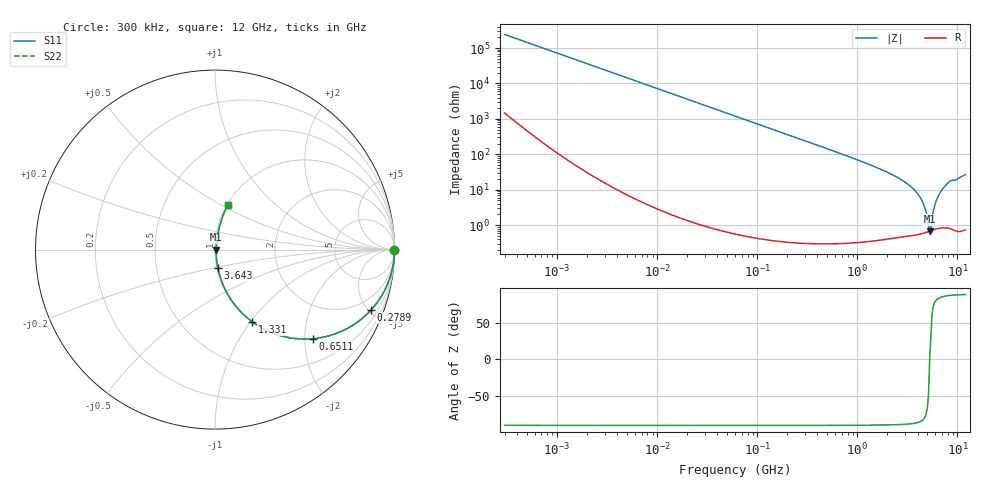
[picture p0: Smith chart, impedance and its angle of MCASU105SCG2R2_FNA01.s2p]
! MCASU105SCG2R2_FNA01  S-PARAMETER MODEL  ( Standard Model )
! Model Generated by TAIYO YUDEN Corporation (http://www.ty-top.com)
! Version 1.0
! TAIYO YUDEN Control No. 230609
! Copyright(c) 2023 TAIYO YUDEN CO.,LTD. All Rights Reserved.
! Product Description (link to TY-COMPAS)
! https://ds.yuden.co.jp/TYCOMPAS/or/detail?pn=MCASU105SCG2R2CFNA01&u=M
! Products Name : Multilayer Ceramic Capacitors
! Characteristics :
!  Capacitance : 2.2 [pF] , Rated Voltage : 50 [V] , TCC : CG / C0G
!  Case Size : 1.0 x 0.5 / 0.039 x 0.02 [mm/inch] , Thickness : 0.5 / 0.02 [mm/inch]
!  (Conditions: Temperature = 25 [degC] , DC Bias Voltage = 0 [V])
! External Node Assignments :
!  1  o---| |---o  2
! GND o---------o GND
! Frequency Range : 0.3MHz  -  12000MHz  [ 401 STEP ]
# MHZ S RI R 50
! Freq[MHz].  S11 Real  S11 Imag  S21 Real  S21 Imag  S12 Real  S12 Imag  S22 Real  S22 Imag
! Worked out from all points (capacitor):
!   401 points, 300 kHz to 12 GHz, reference 50 ohm
!   read as one part in series: C = 2.2 pF near 316.3 kHz
!   lowest |Z| = 674 mohm at 5.279 GHz (marker M1)
!   series resonance near 5.278 GHz, so ESL is about 410 pH
!   S11 on the Smith chart (normalised r, x): 300 kHz: open; 278.9 MHz: 1.01, -5.17; 651.1 MHz: 1.01, -2.19; 1.331 GHz: 1.01, -1.02; 3.643 GHz: 1.01, -0.21; 12 GHz: 1.01, +0.53
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0.3  1 -0.000415  2.68e-06 0.000415  2.68e-06 0.000415  1 -0.000415
1.769972  1 -0.00245  8.24e-06 0.00245  8.24e-06 0.00245  1 -0.00245
10.44266  0.9998 -0.0144  0.000214 0.0144  0.000214 0.0144  0.9998 -0.0144
60  0.9931 -0.0824  0.00687 0.0824  0.00687 0.0824  0.9931 -0.0824
278.9009  0.8697 -0.3361  0.1303 0.3361  0.1303 0.3361  0.8697 -0.3361
353.9943  0.8051 -0.3954  0.1949 0.3954  0.1949 0.3954  0.8051 -0.3954
651.0506  0.5448 -0.4966  0.4552 0.4966  0.4552 0.4966  0.5448 -0.4966
1331.232  0.2073 -0.402  0.7927 0.402  0.7927 0.402  0.2073 -0.402
2088.533  0.0818 -0.2671  0.9182 0.2671  0.9182 0.2671  0.0818 -0.2671
2870.14  0.0347 -0.1705  0.9653 0.1705  0.9653 0.1705  0.0347 -0.1705
3642.919  0.0156 -0.1018  0.9844 0.1018  0.9844 0.1018  0.0156 -0.1018
4158.869  0.00972 -0.0649  0.9903 0.0649  0.9903 0.0649  0.00972 -0.0649
4502.883  0.00766 -0.0431  0.9923 0.0431  0.9923 0.0431  0.00766 -0.0431
4747.894  0.00688 -0.0286  0.9931 0.0286  0.9931 0.0286  0.00688 -0.0286
5140.631  0.00657 -0.00708  0.9934 0.00708  0.9934 0.00708  0.00657 -0.00708
5278.635  0.00669 5.69e-05  0.9933 -5.69e-05  0.9933 -5.69e-05  0.00669 5.69e-05
5565.855  0.00723 0.0129  0.9928 -0.0129  0.9928 -0.0129  0.00723 0.0129
5868.704  0.00841 0.0311  0.9916 -0.0311  0.9916 -0.0311  0.00841 0.0311
6188.031  0.0103 0.05  0.9897 -0.05  0.9897 -0.05  0.0103 0.05
7064.448  0.0184 0.0995  0.9816 -0.0995  0.9816 -0.0995  0.0184 0.0995
8281.503  0.0348 0.1608  0.9652 -0.1608  0.9652 -0.1608  0.0348 0.1608
12000  0.0724 0.2458  0.9276 -0.2458  0.9276 -0.2458  0.0724 0.2458
